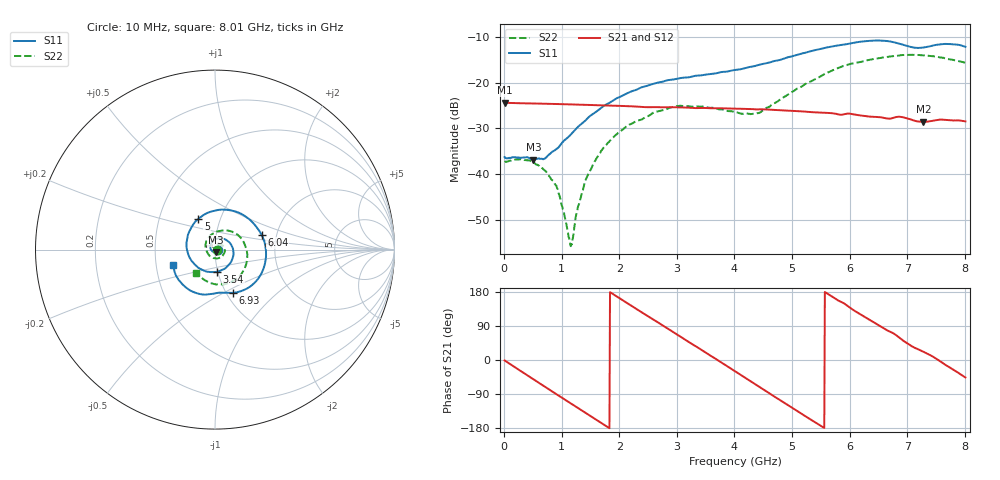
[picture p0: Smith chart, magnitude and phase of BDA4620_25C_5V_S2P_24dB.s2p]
!Agilent Technologies,E5071B,MY42404982,A.09.10
!Date: Wed May 06 09:03:36 2026
!Data & Calibration Information:
!Freq	S11:SOLT2(ON)	S21:SOLT2(ON)	S12:SOLT2(ON)	S22:SOLT2(ON)
# Hz S RI R 50
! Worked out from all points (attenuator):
!   801 points, 10 MHz to 8.01 GHz, reference 50 ohm
!   highest |S21| = -24.40 dB at 10 MHz (marker M1); lowest = -28.6 dB at 7.28 GHz (marker M2)
!   lowest |S11| = -36.9 dB at 510 MHz (marker M3), VSWR 1.03, Z = 50.3 - j1.4 ohm
!   |S11| at or under -10 dB: start of sweep to end of sweep
!   |S22| runs from -55.8 to -13.9 dB; largest |S21 - S12| = 0.00029
!   S11 on the Smith chart (normalised r, x): 10 MHz: 1.03, -0.00; 3.54 GHz: 0.99, -0.25; 5 GHz: 0.79, +0.28; 6.04 GHz: 1.67, +0.30; 6.93 GHz: 1.07, -0.56; 8.01 GHz: 0.62, -0.11
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1e7  0.0153 -0.00107  0.0603 -0.00126  0.0604 -0.0013  0.0135 -0.000464
5.1e8  0.0034 -0.014  0.0374 -0.0459  0.0375 -0.046  0.0123 -0.0054
8.9e8  -0.0165 -0.00821  0.00175 -0.0585  0.0017 -0.0586  0.00418 -0.00641
1.16e9  -0.0253 0.0097  -0.0243 -0.0525  -0.0243 -0.0526  -0.00141 -0.000777
1.19e9  -0.0257 0.0121  -0.0269 -0.0511  -0.0269 -0.0512  -0.00193 0.000134
1.35e9  -0.0249 0.0255  -0.0394 -0.0417  -0.0395 -0.0418  -0.00346 0.005
1.53e9  -0.0176 0.0413  -0.0497 -0.0277  -0.0499 -0.0278  -0.00316 0.0116
1.77e9  0.00212 0.0575  -0.0561 -0.00569  -0.0561 -0.00569  0.00103 0.0207
2.15e9  0.0489 0.0598  -0.0474 0.0286  -0.0474 0.0287  0.0174 0.0293
2.68e9  0.1007 0.0025  -0.00796 0.0534  -0.00791 0.0535  0.0447 0.0191
3.54e9  0.0117 -0.1231  0.0507 0.0143  0.0508 0.0142  0.0352 -0.0404
4.01e9  -0.0978 -0.0976  0.0452 -0.0259  0.0453 -0.026  -0.0109 -0.0467
4.42e9  -0.1567 0.00209  0.0179 -0.0479  0.0179 -0.0479  -0.045 -0.0125
5e9  -0.092 0.1719  -0.0288 -0.0399  -0.029 -0.0399  -0.0314 0.0727
5.35e9  0.0276 0.2222  -0.0446 -0.0166  -0.0447 -0.0167  0.0232 0.1027
6.04e9  0.2593 0.0827  -0.0317 0.0324  -0.0318 0.0325  0.1531 0.054
6.36e9  0.2808 -0.0653  -0.0106 0.0412  -0.0107 0.0411  0.1783 -0.0134
6.68e9  0.2016 -0.2016  0.00954 0.0392  0.00955 0.0394  0.1703 -0.0903
6.93e9  0.1005 -0.2409  0.0262 0.0326  0.0263 0.0326  0.1393 -0.1453
7.28e9  0.00247 -0.2434  0.0347 0.0138  0.0348 0.0138  0.0584 -0.191
7.64e9  -0.1346 -0.2296  0.0386 -0.00721  0.0387 -0.00725  -0.031 -0.1839
8.01e9  -0.2318 -0.0876  0.0262 -0.0272  0.0263 -0.0271  -0.1037 -0.1285
